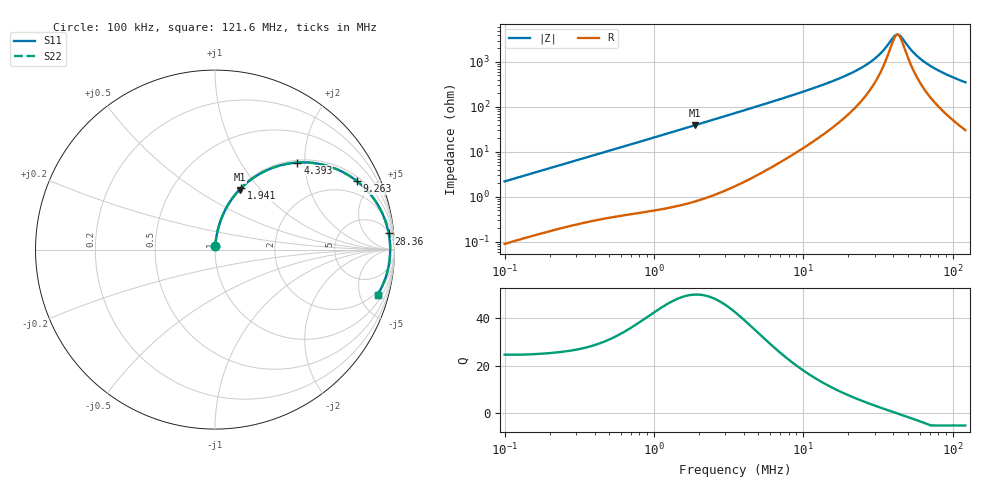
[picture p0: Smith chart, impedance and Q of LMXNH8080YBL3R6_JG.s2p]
! LMXNH8080YBL3R6_JG  S-PARAMETER MODEL  ( General Type )
! Model Generated by TAIYO YUDEN Corporation (https://www.yuden.co.jp/en/)
! Version 1.0
! TAIYO YUDEN Control No. 191025NI43SB-FBB
! Copyright(c) 2019 TAIYO YUDEN CO.,LTD. All Rights Reserved.
! Product Description (link to TY-COMPAS)
! https://ds.yuden.co.jp/TYCOMPAS/or/detail?pn=LMXNH8080YBL3R6NJG&u=M
! Products Name : Inductors
! Characteristics :
!  Inductance : 3.6 uH , SRF(min) : 34 MHz , DC Resistance(max) : 0.0195 Ohm
!  Rated Current : Saturation :6400 mA , Temp Rise : 4900 mA (40 degC)
!  Case Size : 8.0 x 8.0 / 0.315 x 0.315 [mm/inch] , Thickness : 4.2 / 0.165 [mm/inch]
!  (Conditions: Temperature = 25 degC , DC Bias Current/Voltage = 0A / 0V)
! External Node Assignments :
!  1  o---GGG---o  2
! GND o---------o GND
! Frequency Range : 0.1MHz  -  121.638923MHz  [ 402 STEP ]
# MHz S RI R 50
! Freq[MHz].  S11 Real  S11 Imag  S21 Real  S21 Imag  S12 Real  S12 Imag  S22 Real  S22 Imag
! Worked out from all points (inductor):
!   401 points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, 100 kHz to 121.6 MHz, reference 50 ohm
!   read as one part in series: L = 3.47 uH near 103.6 kHz
!   highest Q = 49.7 at 1.873 MHz (marker M1), where L = 3.31 uH
!   self-resonance near 42.67 MHz
!   S11 on the Smith chart (normalised r, x): 100 kHz: 1.00, +0.04; 1.941 MHz: 1.02, +0.81; 4.393 MHz: 1.05, +1.84; 9.263 MHz: 1.21, +4.02; 28.36 MHz: 6, +20; 121.6 MHz: 1.61, -7.02
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0.1  0.00137 0.0219  0.9986 -0.0219  0.9986 -0.0219  0.00137 0.0219
0.328662  0.00739 0.0692  0.9926 -0.0692  0.9926 -0.0692  0.00739 0.0692
1.080188  0.0526 0.212  0.9474 -0.212  0.9474 -0.212  0.0526 0.212
1.873236  0.1366 0.3335  0.8634 -0.3335  0.8634 -0.3335  0.1366 0.3335
1.940965  0.145 0.3422  0.855 -0.3422  0.855 -0.3422  0.145 0.3422
3.550168  0.3576 0.4675  0.6424 -0.4675  0.6424 -0.4675  0.3576 0.4675
4.393404  0.4594 0.485  0.5406 -0.485  0.5406 -0.485  0.4594 0.485
6.156616  0.6247 0.4669  0.3753 -0.4669  0.3753 -0.4669  0.6247 0.4669
9.262618  0.7899 0.3825  0.2101 -0.3825  0.2101 -0.3825  0.7899 0.3825
11.46267  0.8518 0.3246  0.1482 -0.3246  0.1482 -0.3246  0.8518 0.3246
19.52839  0.9417 0.1796  0.0583 -0.1796  0.0583 -0.1796  0.9417 0.1796
24.16677  0.9592 0.127  0.0408 -0.127  0.0408 -0.127  0.9592 0.127
28.3552  0.9677 0.0898  0.0323 -0.0898  0.0323 -0.0898  0.9677 0.0898
33.26954  0.9731 0.054  0.0269 -0.054  0.0269 -0.054  0.9731 0.054
37.67347  0.9754 0.0269  0.0246 -0.0269  0.0246 -0.0269  0.9754 0.0269
41.17172  0.9761 0.00769  0.0239 -0.00769  0.0239 -0.00769  0.9761 0.00769
43.42472  0.9761 -0.0038  0.0239 0.0038  0.0239 0.0038  0.9761 -0.0038
45.80101  0.9759 -0.0153  0.0241 0.0153  0.0241 0.0153  0.9759 -0.0153
54.70184  0.9732 -0.054  0.0268 0.054  0.0268 0.054  0.9732 -0.054
65.33242  0.9671 -0.0938  0.0329 0.0938  0.0329 0.0938  0.9671 -0.0938
86.80238  0.9486 -0.1616  0.0514 0.1616  0.0514 0.1616  0.9486 -0.1616
121.6389  0.907 -0.2504  0.093 0.2504  0.093 0.2504  0.907 -0.2504
